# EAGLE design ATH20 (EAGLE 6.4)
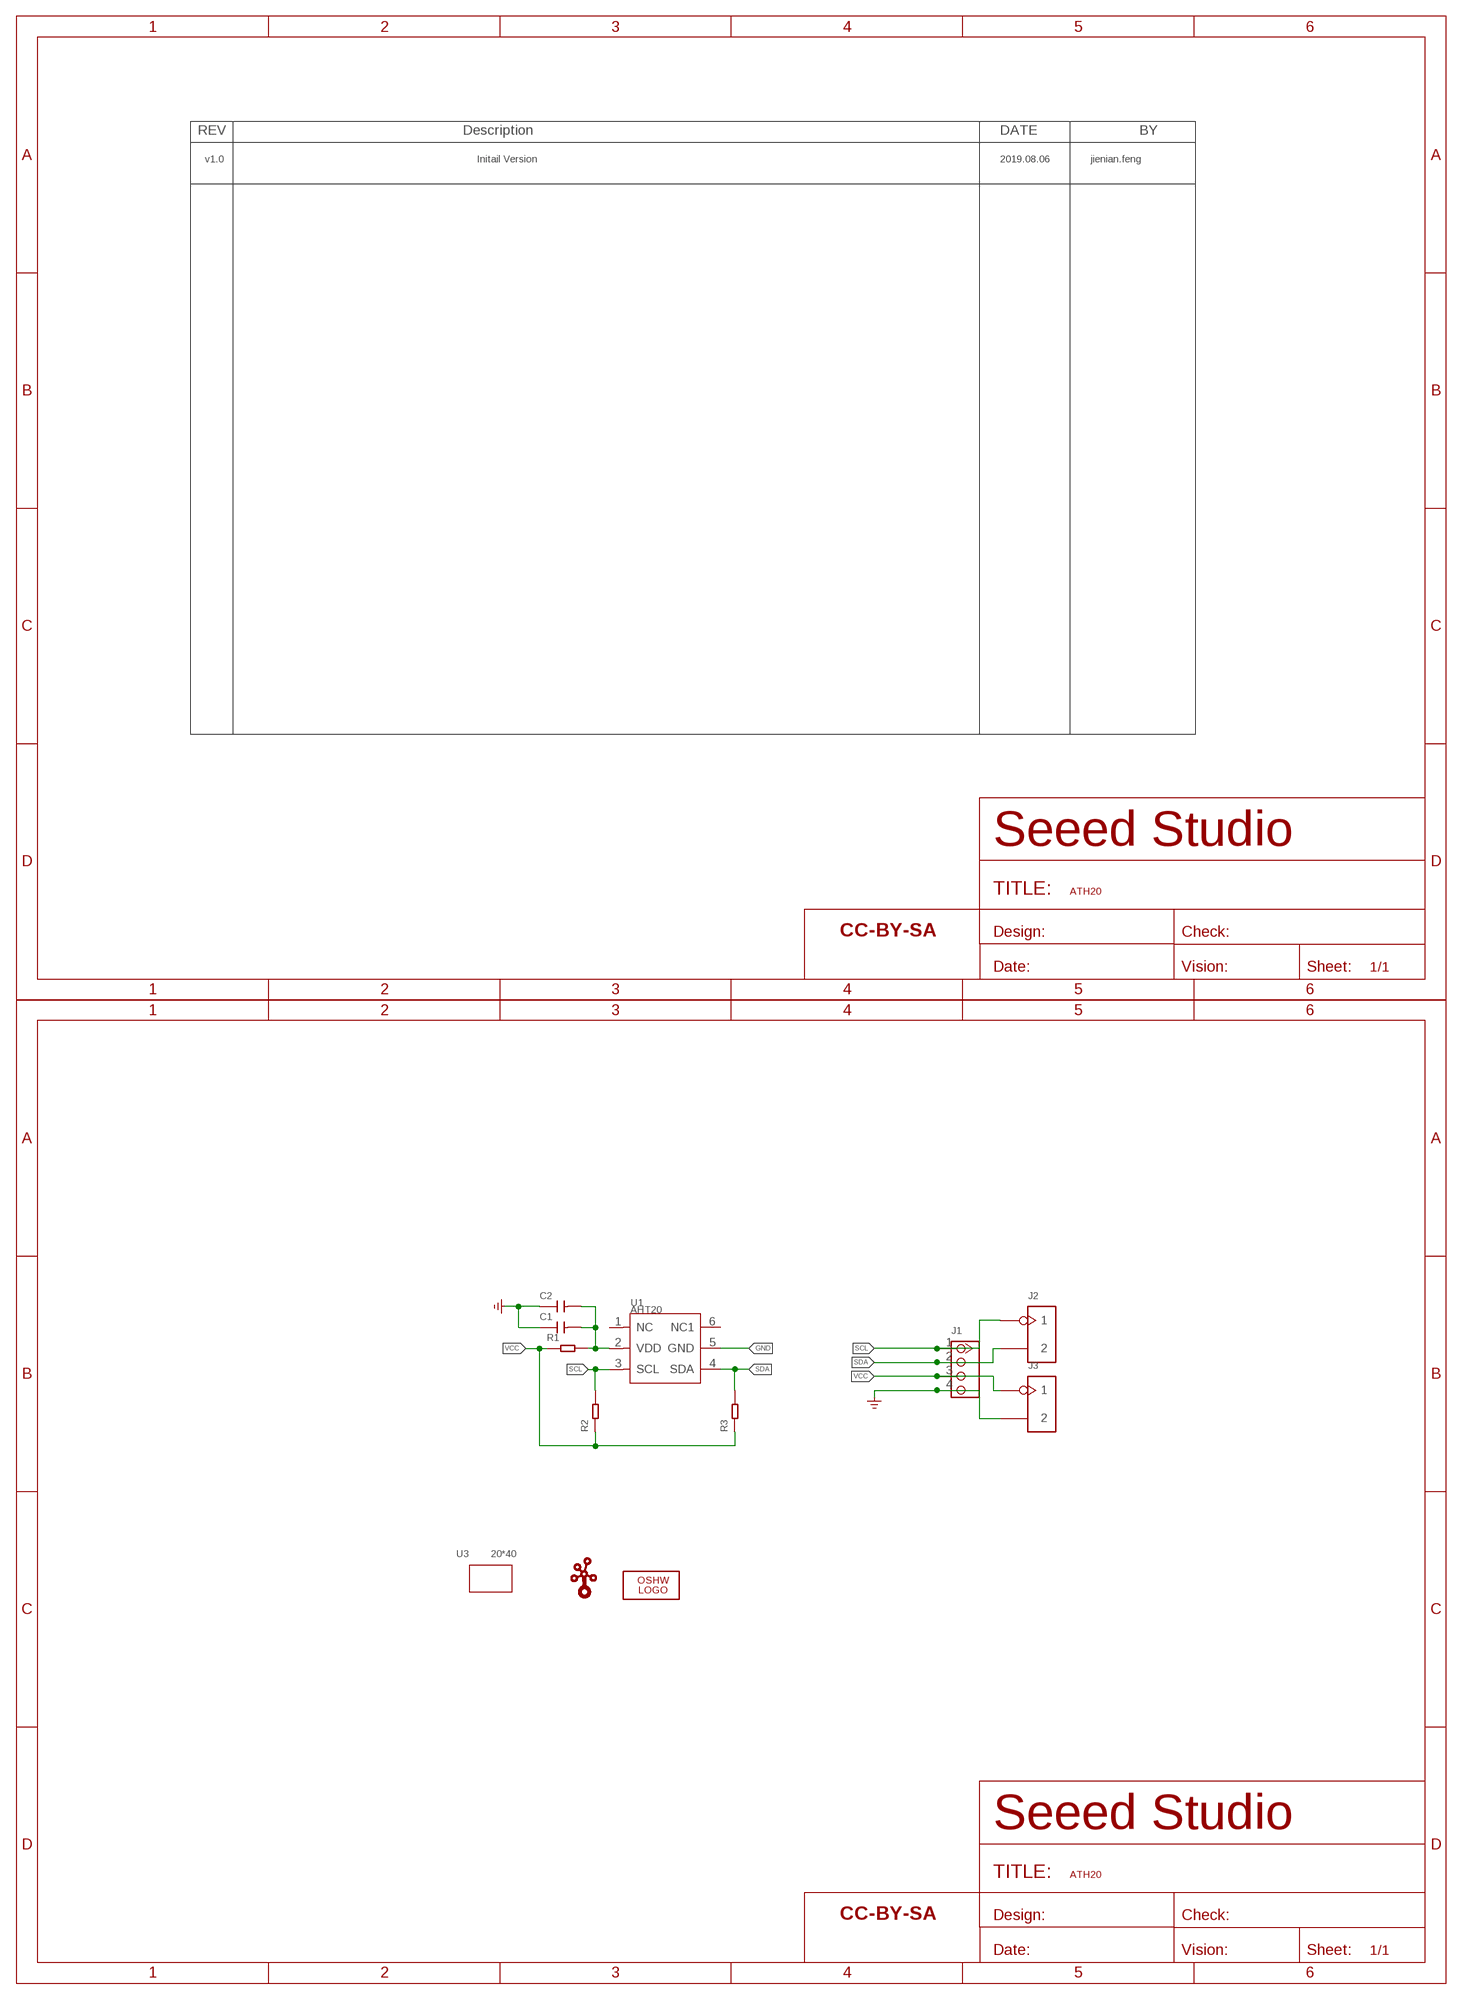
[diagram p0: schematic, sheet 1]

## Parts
C1  CAP-0603  [C0603]
C2  CAP-0603  [C0603]
FR1  SEEEDSTUDIO-OPEN-SCH-FRAME  [SEEEDSTUDIO-PCB-FRAME]
FR2  SEEEDSTUDIO-OPEN-SCH-FRAME  [SEEEDSTUDIO-PCB-FRAME]
J1  GROVE-CONNECTOR-DIP-320110033  [HW4-2.0]
J2  HEADER-2P-2.54  [H2P-2.54-80/50MIL]
J3  HEADER-2P-2.54  [H2P-2.54-80/50MIL]
LOGO1  LOGO-OSHW-FILLX0150-NT  [OSHW_FILLX150_NOTEXT]
R1  RES-0603  [R0603]
R2  RES-0603  [R0603]
R3  RES-0603  [R0603]
U1  AHT20  SENSOR-AHT20  [SNR6-1.0-3X3X1MM]
U3  20*40  GROVE-1X1-TOP  [GROVE-1X1-TEST-PLATFORM-TOP]
U$1  LOGO-GROVETWIGLOGO_SMALL  [GROVE-SILK-SMALL]

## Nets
GND: C1.1 C2.1 J1.4 J3.2 U1.5(GND) ; supply symbol labelled GND_POWER
N$1: C1.2 C2.2 R1.2 U1.2(VDD)
SCL: J1.1 J2.1 R2.2 U1.3(SCL)
SDA: J1.2 J2.2 R3.2 U1.4(SDA)
VCC: J1.3 J3.1 R1.1 R2.1 R3.1
Unconnected: U1.1(NC) U1.6(NC1)

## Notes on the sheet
- v1.0 | Initail Version | 2019.08.06 | jienian.feng

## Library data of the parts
C1 C2 = Discrete-new:CAP: Ceramic Capacitors
FR1 FR2 = moudle-new:SEEEDSTUDIO-OPEN-SCH-FRAME
J1 = Connector-new:GROVE-CONNECTOR-DIP
J2 J3 = Connector-new:HEADER-2P
LOGO1 = logo:LOGO-OSHW-FILL; PARTNO: DNP
R1-R3 = Discrete-new:RES
U1 = Longan-IC:SENSOR-AHT20
U3 = moudle-new:GROVE
U$1 = logo:LOGO-GROVE; PARTNO: DNP

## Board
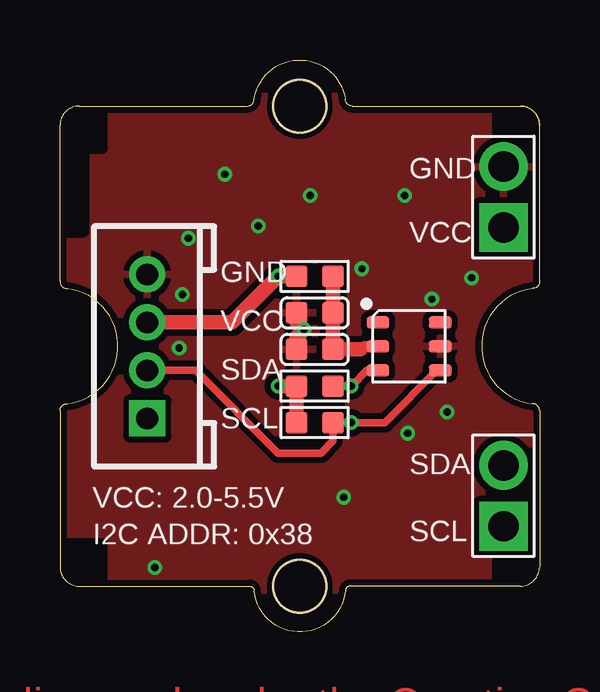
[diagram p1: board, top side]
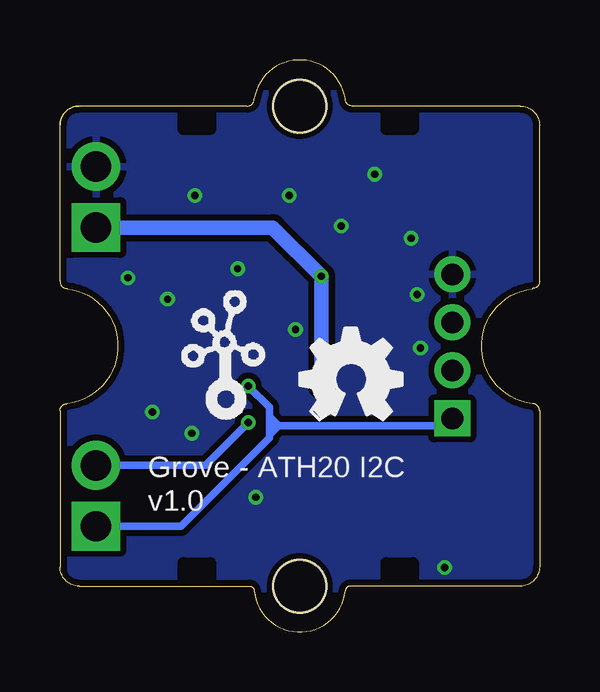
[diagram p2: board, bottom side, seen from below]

Size 20 x 23.83 mm. Coordinates in mm from the lower left corner, seen from the top.
Copper layers (1*16): Top 0.035mm / dielectric 1.5mm / Bottom 0.035mm
Design rules "SeeedStudio_2layer_DRU_no_angle_20140221 *": minimum track width 1mil, minimum drill 10mil, track to track 6mil, track to pad 6mil, pad to pad 6mil, via to via 6mil, smd to smd 0mil, copper to edge 10mil, drill to drill 10mil, minimum pad ring 4mil, minimum via ring 4mil, stop-mask expansion 2mil, vias tented up to drill 25mil, thermal gap 10mil

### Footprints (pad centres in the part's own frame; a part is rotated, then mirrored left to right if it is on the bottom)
C0603 = smd 0.889 x 0.889: 1 -0.762,0; 2 0.762,0
HW4-2.0 = drill 0.9 pad 1.5 square: 1 -3,0 | drill 0.9 pad 1.5: 2 -1,0; 3 1,0; 4 3,0
H2P-2.54-80/50MIL = drill 1.27 pad 2.032 square: 1 0,1.27 | drill 1.27 pad 2.032: 2 0,-1.27
R0603 = smd 0.889 x 0.889: 1 -0.762,0; 2 0.762,0
SNR6-1.0-3X3X1MM = smd 0.95 x 0.5: 1 -1.3,1; 2 -1.3,0; 3 -1.3,-1; 4 1.3,-1; 5 1.3,0; 6 1.3,1
GROVE-1X1-TEST-PLATFORM-TOP = hole 2.2: 9.987,0.013; -10.013,0.013

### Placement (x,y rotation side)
C1  10.62,13.29 0 top
C2  10.62,11.77 0 top
FR1  not placed on the board
FR2  not placed on the board
J1  3.64,11.9 90 top
J2  18.5,5.67 180 top
J3  18.5,18.12 180 top
LOGO1  9.99,8.85 0 bottom
R1  10.62,14.82 0 top
R2  10.62,10.24 0 top
R3  10.62,8.72 0 top
U1  14.56,11.9 0 top
U3  9.99,11.9 270 top
U$1  15.32,8.72 0 bottom

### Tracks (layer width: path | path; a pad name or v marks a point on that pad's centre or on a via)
GND  (via drill 0.3 pad 0.61)
  Top 0.61: C2.1 9.86,12.28 v10.18,12.59 9.86,12.91 C1.1
  other vias: 8.27,16.91 5.35,16.4 15.51,13.86 10.43,18.18 6.88,19.07 12.59,15.13 16.15,9.16 14.5,8.28 11.83,5.61 3.95,2.69 14.37,18.18 17.16,14.75 4.97,11.83 5.1,14.05
  pour Bottom (isolate 0.254, rank 6): -0.17,22.44 -0.17,1.74 20.4,1.74 20.4,22.44
  pour Top (isolate 0.254, rank 6): 20.4,22.31 -0.17,22.31 -0.17,1.74 20.4,1.74
N$1
  Top 0.406: U1.2 12.65,11.9 12.53,11.77
  Top 0.61: R1.2 C1.2 C2.2 12.53,11.77
SCL  (via drill 0.3 pad 0.61)
  Top 0.305: R2.2 v12.15,10.24 12.8,10.9 U1.3
  Bottom 0.305: 11.26,8.21 11.26,8.59 | 11.26,8.59 11.26,8.97 | 11.26,8.97 11.26,9.36 v12.15,10.24 | 10.88,8.59 11.26,8.59 | 10.88,8.59 11.26,8.97 | 10.88,8.59 11.26,8.21 | 10.88,8.59 3.94,8.59 J1.1 | J2.1 14.94,4.4 11.26,8.09 11.26,8.21
SDA  (via drill 0.3 pad 0.61)
  Top 0.305: U1.4 15.72,10.9 13.54,8.72 v12.15,8.72 R3.2 11.38,7.96 10.88,7.45 9.1,7.45 5.65,10.9 J1.2
  Bottom 0.305: J2.2 13.92,6.94 v12.15,8.72
VCC  (via drill 0.3 pad 0.61)
  Top 0.61: v9.1,10.24 R2.1 R3.1 | R1.1 v9.1,14.82 7.18,12.9 J1.3
  Bottom 0.61: v9.1,10.24 v9.1,14.82 11.13,16.85 J3.1

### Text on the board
tPlace: VCC: 2.0-5.5V | I2C ADDR: 0x38
tNames: GND | VCC | GND | VCC | SDA | SCL | SDA | SCL
bNames: Grove - ATH20 I2C | v1.0

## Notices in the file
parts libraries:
moudle-new: This work is licensed under the Creative Commons Attribution 4.0 International License.
To view a copy of this license,visit:
http://creativecommons.org/licenses/by-sa/4.0
moudle-new: CC-BY-SA
